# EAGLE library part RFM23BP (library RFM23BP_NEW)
RFM23BP module by HopeRF
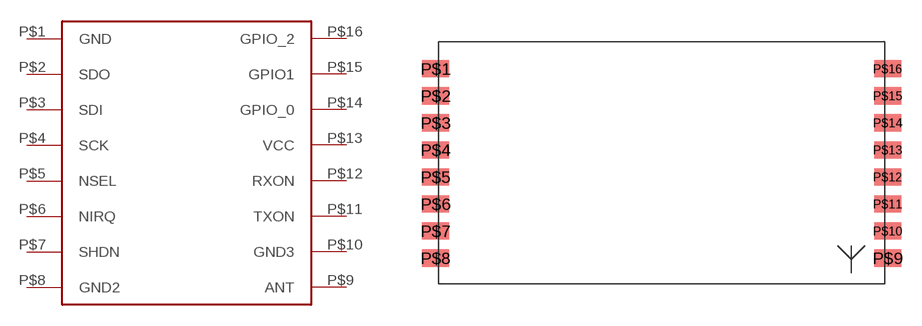
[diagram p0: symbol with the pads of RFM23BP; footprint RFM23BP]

Designator prefix -

## RFM23BP  [RFM23BP]
P$1  GND
P$2  SDO
P$3  SDI
P$4  SCK
P$5  NSEL
P$6  NIRQ
P$7  SHDN
P$8  GND2
P$9  ANT
P$10  GND3
P$11  TXON
P$12  RXON
P$13  VCC
P$14  GPIO_0
P$15  GPIO1
P$16  GPIO_2

## Footprint RFM23BP (pad centres in mm)
smd 2 x 1.27: P$1 -16.7,7.1; P$2 -16.7,5.1; P$3 -16.7,3.1; P$4 -16.7,1.1; P$5 -16.7,-0.9; P$6 -16.7,-2.9; P$7 -16.7,-4.9; P$8 -16.7,-6.9; P$9 16.7,-6.9; P$10 16.7,-4.9; P$11 16.7,-2.9; P$12 16.7,-0.9; P$13 16.7,1.1; P$14 16.7,3.1; P$15 16.7,5.1; P$16 16.7,7.1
